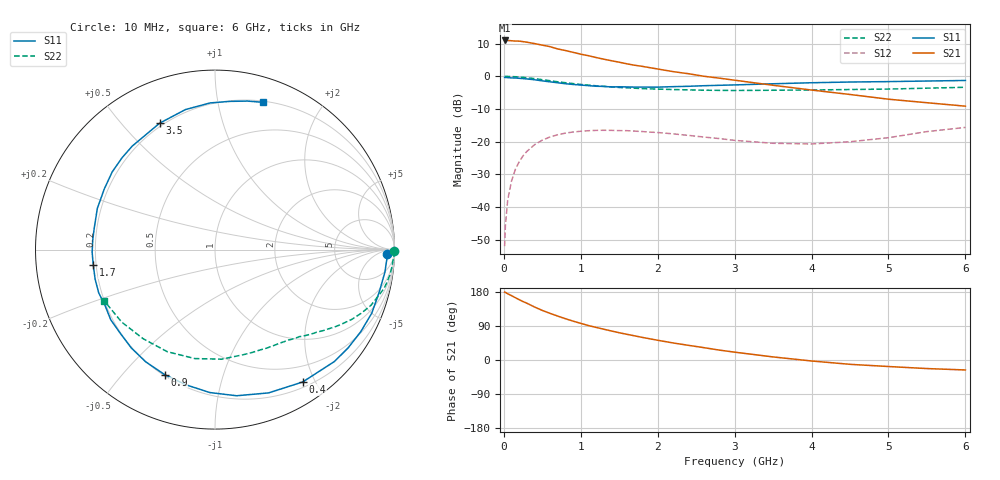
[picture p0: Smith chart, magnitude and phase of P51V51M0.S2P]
! SIEMENS Small Signal Semiconductors
! BFP183
! Si NPN RF Bipolar Junction Transistor in SOT143
! VCE = 1.5 V  IC = 1 mA
! Common Emitter S-Parameters:  March  1996
# GHz  S  MA  R  50
!  f  S11  S21  S12  S22
! GHz  MAG  ANG  MAG  ANG  MAG  ANG  MAG  ANG
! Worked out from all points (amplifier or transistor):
!   36 points, 10 MHz to 6 GHz, reference 50 ohm
!   highest |S21| = 11.0 dB at 10 MHz (marker M1)
!   |S21| within 3 dB of that: start of sweep to 783.8 MHz
!   unconditionally stable (mu >= 1): 2.443 GHz to end of sweep
!   at 250 MHz: K = 0.10, MSG = 17.5 dB, |S12| = -24.4 dB
!   at 1.4 GHz: K = 0.56, MSG = 10.7 dB, |S12| = -16.6 dB
!   at 6 GHz: K = 1.09, MAG = 1.4 dB, |S12| = -15.7 dB
!   S11 on the Smith chart (normalised r, x): 10 MHz: 36, -22; 400 MHz: 0.27, -1.83; 900 MHz: 0.21, -0.65; 1.7 GHz: 0.19, -0.06; 3.5 GHz: 0.19, +0.64; 6 GHz: 0.21, +1.36
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0.01  0.9606 -1.4  3.543 179.3  0.0025 87.1  0.9999 -0.5
0.02  0.9595 -2.8  3.532 178.6  0.0051 84.3  0.9997 -1.1
0.05  0.9549 -7.6  3.537 174.8  0.0127 87.2  0.9951 -2.6
0.1  0.9452 -14.5  3.507 169.7  0.0249 80.1  0.9908 -5.4
0.15  0.9425 -22.1  3.468 164.4  0.0376 76.1  0.9851 -8.0
0.2  0.9321 -29.4  3.459 159.2  0.0493 72.6  0.9764 -10.5
0.25  0.922 -36.4  3.398 154.1  0.0605 68.0  0.9655 -13.1
0.4  0.8847 -56.5  3.171 139.8  0.0897 56.2  0.9224 -19.7
0.5  0.8524 -69.5  3.003 130.8  0.1053 49.0  0.8879 -23.6
0.6  0.8231 -81.6  2.848 123.1  0.1177 42.5  0.8559 -27.0
0.7  0.7969 -92.1  2.627 115.9  0.1273 36.7  0.8245 -29.9
0.9  0.7508 -112.0  2.33 102.6  0.1402 27.0  0.7737 -34.7
1.1  0.7195 -130.4  2.068 90.9  0.1468 18.8  0.7314 -38.9
1.4  0.6873 -152.9  1.732 76.5  0.1486 8.9  0.6886 -44.5
1.7  0.6838 -172.7  1.478 63.8  0.1447 1.8  0.6574 -49.5
1.9  0.6832 175.6  1.356 55.9  0.1397 -1.9  0.6423 -52.9
2.2  0.6946 160.7  1.18 45.0  0.1314 -6.1  0.6274 -58.2
2.8  0.7281 135.3  0.938 26.2  0.1113 -9.0  0.6092 -70.3
3.5  0.7688 113.7  0.729 8.1  0.0942 -2.7  0.6116 -86.6
4.5  0.8177 91.9  0.527 -11.4  0.0995 16.0  0.6278 -115.0
5.5  0.8469 77.7  0.394 -22.6  0.1423 23.3  0.6584 -142.2
6  0.8636 71.8  0.349 -26.3  0.1649 20.7  0.6795 -155.0
